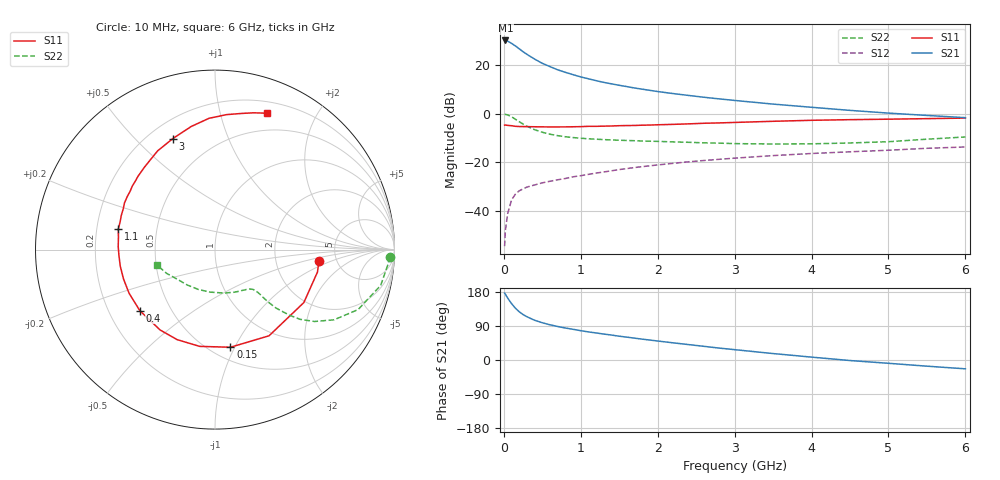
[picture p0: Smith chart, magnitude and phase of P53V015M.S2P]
! SIEMENS Small Signal Semiconductors
! BFP183
! Si NPN RF Bipolar Junction Transistor in SOT143
! VCE = 3 V  IC = 15 mA
! Common Emitter S-Parameters:  March  1996
# GHz  S  MA  R  50
!  f  S11  S21  S12  S22
! GHz  MAG  ANG  MAG  ANG  MAG  ANG  MAG  ANG
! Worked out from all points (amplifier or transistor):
!   36 points, 10 MHz to 6 GHz, reference 50 ohm
!   highest |S21| = 30.1 dB at 20 MHz (marker M1)
!   |S21| within 3 dB of that: start of sweep to 181.7 MHz
!   unconditionally stable (mu >= 1): 945.8 MHz to 5.587 GHz
!   at 250 MHz: K = 0.41, MSG = 28.2 dB, |S12| = -30.9 dB
!   at 1.4 GHz: K = 1.12, MAG = 15.8 dB, |S12| = -23.5 dB
!   at 6 GHz: K = 0.96, MSG = 6.0 dB, |S12| = -13.7 dB
!   S11 on the Smith chart (normalised r, x): 10 MHz: 3.65, -0.71; 150 MHz: 0.62, -0.96; 400 MHz: 0.33, -0.32; 1.1 GHz: 0.29, +0.10; 3 GHz: 0.29, +0.65; 6 GHz: 0.31, +1.40
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0.01  0.583 -6.3  31.86 176.6  0.0019 88.5  0.9762 -2.4
0.02  0.5844 -12.4  32 173.5  0.004 78.6  0.9673 -4.9
0.05  0.5763 -30.8  30.98 163.3  0.0089 79.5  0.9444 -12.2
0.1  0.5668 -57.9  27.88 148.9  0.0169 65.9  0.8648 -22.7
0.15  0.5508 -81.0  24.69 136.8  0.0222 58.9  0.7705 -30.5
0.2  0.5459 -99.0  21.55 127.3  0.0261 54.0  0.6847 -35.8
0.25  0.5442 -112.8  18.76 119.9  0.0285 50.1  0.6135 -39.3
0.3  0.5423 -124.3  16.6 114.2  0.0311 48.1  0.5527 -41.4
0.4  0.5396 -140.9  13.24 104.9  0.0344 46.7  0.4694 -43.8
0.5  0.5369 -153.1  10.85 98.3  0.038 45.8  0.4161 -44.6
0.6  0.5353 -162.3  9.282 92.9  0.041 46.2  0.3796 -44.8
0.7  0.5358 -170.1  7.984 88.4  0.0439 47.1  0.3541 -44.8
0.9  0.5395 178.2  6.339 81.0  0.0506 48.0  0.3235 -45.3
1.1  0.551 168.0  5.212 74.1  0.0568 49.1  0.3051 -46.5
1.5  0.5675 152.7  3.835 62.8  0.0712 49.5  0.2852 -50.7
1.8  0.5812 142.4  3.19 55.0  0.0817 48.6  0.2749 -55.4
2.2  0.6043 130.6  2.594 45.3  0.0956 46.6  0.2635 -63.0
3  0.6619 110.8  1.874 27.3  0.1222 40.9  0.2431 -82.3
3.5  0.6987 100.9  1.576 17.0  0.1379 36.9  0.2385 -96.6
4.5  0.7547 85.1  1.171 -1.4  0.1651 28.5  0.2506 -128.1
5.5  0.7921 74.2  0.922 -16.3  0.1948 20.9  0.2995 -153.6
6  0.8129 69.2  0.829 -23.3  0.2074 16.4  0.3328 -164.6
